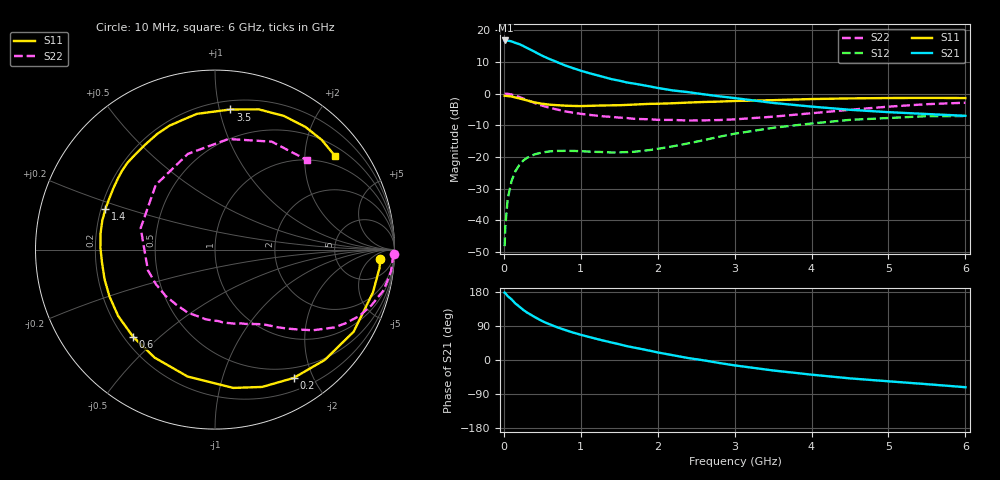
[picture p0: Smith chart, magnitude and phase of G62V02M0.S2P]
! SIEMENS Small Signal Semiconductors
! BFG193
! Si NPN RF Bipolar Junction Transistor in SOT223
! VCE = 2 V  IC = 2 mA
! Common Emitter S-Parameters:  August  1996
# GHz  S  MA  R  50
!  f  S11  S21  S12  S22
! GHz  MAG  ANG  MAG  ANG  MAG  ANG  MAG  ANG
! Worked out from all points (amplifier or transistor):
!   36 points, 10 MHz to 6 GHz, reference 50 ohm
!   highest |S21| = 16.8 dB at 20 MHz (marker M1)
!   |S21| within 3 dB of that: start of sweep to 353.5 MHz
!   unconditionally stable (mu >= 1): 1.366 GHz to 2.702 GHz
!   at 250 MHz: K = 0.18, MSG = 18.1 dB, |S12| = -21.2 dB
!   at 1.4 GHz: K = 1.03, MAG = 10.5 dB, |S12| = -18.6 dB
!   at 6 GHz: K = 0.98, MSG = 0.1 dB, |S12| = -7.1 dB
!   S11 on the Smith chart (normalised r, x): 10 MHz: 17, -11; 200 MHz: 0.36, -1.73; 600 MHz: 0.24, -0.41; 1.4 GHz: 0.22, +0.17; 3.5 GHz: 0.27, +1.08; 6 GHz: 0.74, +2.74
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0.01  0.9219 -3.2  6.857 177.7  0.0039 90.0  0.995 -1.5
0.02  0.9224 -6.4  6.88 176.5  0.0082 87.5  0.9919 -2.7
0.05  0.9117 -15.2  6.853 168.7  0.0217 80.9  0.9884 -6.9
0.1  0.8977 -30.6  6.658 160.0  0.0416 73.6  0.9669 -13.5
0.15  0.8673 -45.1  6.308 149.2  0.0595 64.7  0.9252 -19.6
0.2  0.8386 -58.5  6.026 141.1  0.0741 58.2  0.885 -24.7
0.25  0.8092 -71.0  5.65 132.6  0.087 51.4  0.8345 -29.5
0.3  0.7775 -82.4  5.251 125.5  0.0965 46.4  0.7924 -33.2
0.4  0.7235 -102.2  4.562 113.5  0.1097 37.6  0.7079 -39.4
0.5  0.6896 -119.2  3.937 102.5  0.1174 30.5  0.6421 -43.9
0.6  0.6662 -133.3  3.484 93.8  0.1223 25.7  0.5943 -47.7
0.7  0.6542 -145.5  3.104 85.9  0.1243 22.1  0.5559 -51.1
0.8  0.6432 -156.1  2.768 78.9  0.1246 19.1  0.5228 -54.1
1.1  0.6385 179.1  2.113 61.2  0.1213 15.2  0.4619 -63.8
1.4  0.6513 159.7  1.686 46.2  0.1174 15.8  0.428 -74.7
1.6  0.6614 148.9  1.495 36.5  0.1191 18.8  0.4104 -83.1
2.2  0.7022 123.8  1.118 12.5  0.1471 27.1  0.3832 -112.9
2.8  0.746 103.4  0.904 -7.9  0.2079 25.4  0.3817 -149.9
3.5  0.7855 83.7  0.711 -27.6  0.2877 11.3  0.4312 163.8
4.5  0.8379 62.7  0.554 -48.5  0.3842 -12.1  0.5543 105.8
5.5  0.8528 45.8  0.475 -63.8  0.4394 -39.7  0.6793 62.3
6  0.8484 37.8  0.445 -71.8  0.4398 -54.5  0.7161 44.0
